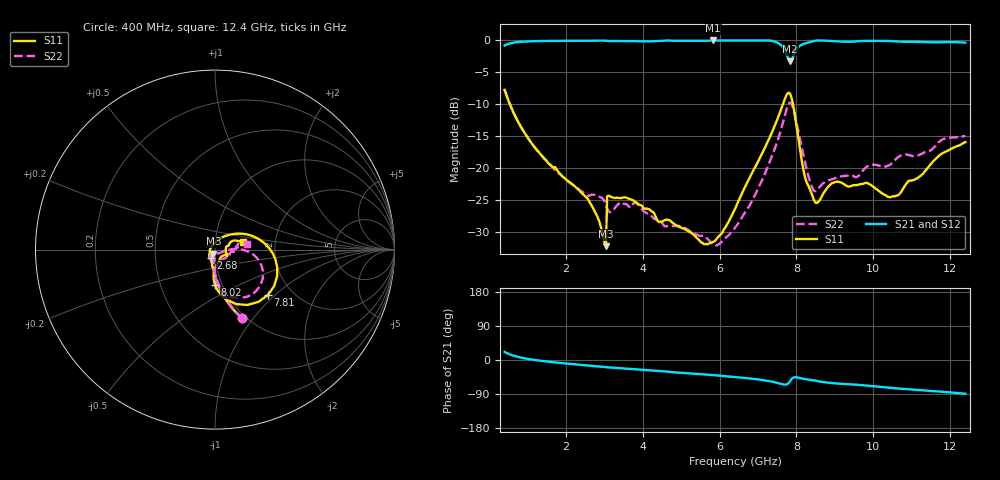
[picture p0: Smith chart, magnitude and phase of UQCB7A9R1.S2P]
!  Part Number  UQCB7A9R1	Mounting Orientation: Vertical
!  Description: RF capacitors
!  Application: Coupling, Bypass, Tuning, DC Block
!  Filters, Matching
# GHZ S DB R 50
! Freq  |S11|  S11 Ph  |S21|  S21 Ph  |S12|  S12 Ph  |S22|  S22 Ph
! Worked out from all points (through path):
!   401 points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, 400 MHz to 12.4 GHz, reference 50 ohm
!   highest |S21| = 0.00 dB at 5.83 GHz (marker M1); lowest = -3.2 dB at 7.84 GHz (marker M2)
!   group delay of S21, straight-line fit = 21.6 ps
!   lowest |S11| = -32.3 dB at 3.04 GHz (marker M3), VSWR 1.05, Z = 49.1 - j2.22 ohm
!   |S11| at or under -10 dB: 537 MHz to 7.648 GHz (7.111 GHz wide, 174 % of centre); 7.91 GHz to end of sweep
!   |S22| runs from -32.2 to -7.7 dB; largest |S21 - S12| = 0.0043
!   S11 on the Smith chart (normalised r, x): 400 MHz: 0.96, -0.88; 2.68 GHz: 0.95, -0.08; 7.81 GHz: 1.51, -0.90; 8.02 GHz: 0.93, -0.38; 12.4 GHz: 1.36, +0.12
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0.4  -7.74 -68.7  -0.81 21.4  -0.82 21.5  -7.73 -68.2
1.18  -16.74 -90.0  -0.11 0.2  -0.13 0.2  -16.75 -88.5
2.41  -23.95 -109.4  -0.04 -13.1  -0.06 -13.0  -23.67 -96.2
2.68  -26.08 -117.3  -0.05 -15.4  -0.06 -15.3  -24.17 -93.8
2.98  -31.16 -119.3  -0.01 -18.2  -0.03 -18.1  -25.00 -101.7
3.04  -32.27 -111.7  -0.03 -18.8  -0.05 -18.8  -25.89 -105.9
3.13  -24.39 -106.0  -0.09 -19.6  -0.10 -19.5  -26.91 -111.4
3.82  -25.39 -123.7  -0.11 -25.0  -0.13 -25.0  -25.51 -122.0
4.42  -28.49 -135.3  -0.08 -28.9  -0.09 -28.8  -28.46 -124.8
5.83  -31.61 139.7  0.00 -39.9  -0.01 -39.8  -31.96 -78.9
6.4  -26.42 80.7  -0.01 -45.0  -0.01 -44.8  -29.35 -31.3
7.45  -13.15 20.4  -0.21 -59.1  -0.20 -59.0  -16.76 0.2
7.63  -10.30 0.6  -0.94 -63.8  -0.93 -63.6  -13.29 -7.7
7.81  -8.21 -40.6  -3.11 -59.2  -3.10 -59.1  -9.83 -38.4
7.84  -8.43 -50.1  -3.25 -55.0  -3.24 -54.8  -9.74 -46.7
8.02  -14.13 -90.0  -1.25 -46.0  -1.24 -45.9  -13.39 -83.5
8.2  -20.86 -86.5  -0.51 -50.0  -0.50 -49.8  -18.47 -89.8
8.41  -24.26 -65.8  -0.14 -53.2  -0.12 -53.0  -23.10 -70.8
8.56  -25.39 -42.8  -0.01 -55.9  -0.01 -55.8  -23.29 -48.2
9.07  -22.14 -27.9  -0.14 -62.1  -0.13 -62.0  -21.43 -28.0
10.42  -24.59 -5.8  -0.08 -73.2  -0.06 -73.1  -19.57 3.4
12.4  -15.94 16.0  -0.34 -89.2  -0.32 -89.2  -14.95 9.8
